VAR_GLOBAL
	BUS_OUTPUT	AT %Q*:  ARRAY[1..2] OF ARRAY[0..253]  OF BYTE;	(* 1. ARRAY = Number of antennas; 2. ARRAY = I/O Length *)
    BUS_INPUT	AT %I*:  ARRAY[1..2] OF ARRAY[0..253]  OF BYTE;	(* 1. ARRAY = Number of antennas; 2. ARRAY = I/O Length *)	
END_VAR
